FUNCTION FC 20 : VOID
TITLE =RICEZIONE DATI DAL PLC_LINE
AUTHOR : Esposito
FAMILY : EGAL_srl
NAME : COM_MPI
VERSION : 0.1


VAR_TEMP
  VALUE_OPSCHUIF : DINT ;
END_VAR
BEGIN
NETWORK
TITLE =COMMAND FOR SFC66
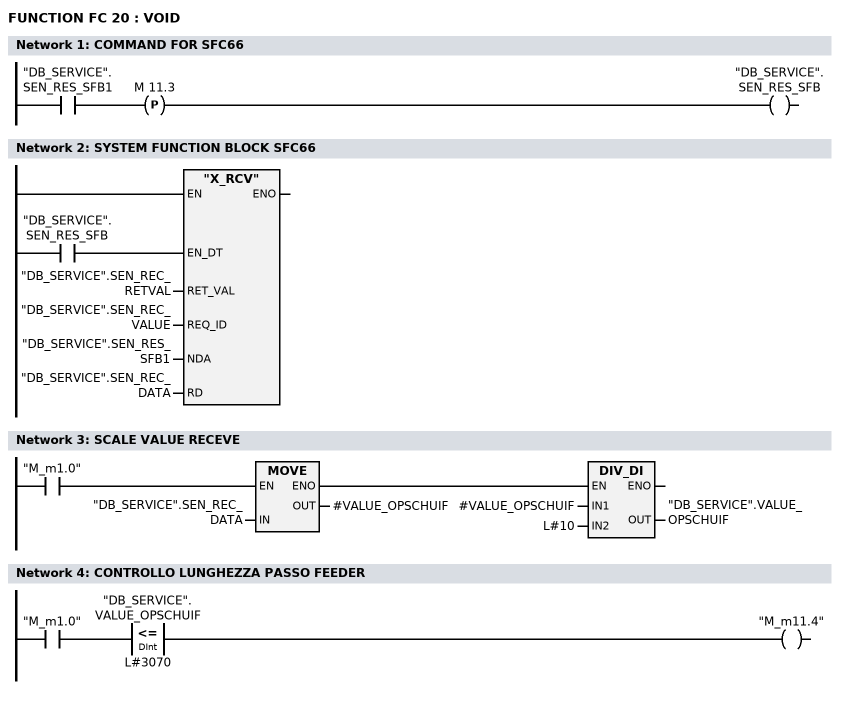
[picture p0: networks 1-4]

      U     "DB_SERVICE".SEN_RES_SFB1;
      FP    M     11.3;
      =     "DB_SERVICE".SEN_RES_SFB;
NETWORK
TITLE =SYSTEM FUNCTION BLOCK SFC66

      U     "DB_SERVICE".SEN_RES_SFB;
      =     L      4.0;
      BLD   103;
      CALL "X_RCV" (
           EN_DT                    := L      4.0,
           RET_VAL                  := "DB_SERVICE".SEN_REC_RETVAL,
           REQ_ID                   := "DB_SERVICE".SEN_REC_VALUE,
           NDA                      := "DB_SERVICE".SEN_RES_SFB1,
           RD                       := "DB_SERVICE".SEN_REC_DATA);
      NOP   0;
NETWORK
TITLE =SCALE VALUE RECEVE

      U(    ;
      U     "M_m1.0";
      SPBNB _001;
      L     "DB_SERVICE".SEN_REC_DATA;
      T     #VALUE_OPSCHUIF;
      SET   ;
      SAVE  ;
      CLR   ;
_001: U     BIE;
      )     ;
      SPBNB _002;
      L     #VALUE_OPSCHUIF;
      L     L#10;
      /D    ;
      T     "DB_SERVICE".VALUE_OPSCHUIF;
_002: NOP   0;
NETWORK
TITLE =CONTROLLO LUNGHEZZA PASSO FEEDER

      U     "M_m1.0";
      U(    ;
      L     "DB_SERVICE".VALUE_OPSCHUIF;
      L     L#3070;
      <=D   ;
      )     ;
      =     "M_m11.4";
END_FUNCTION

